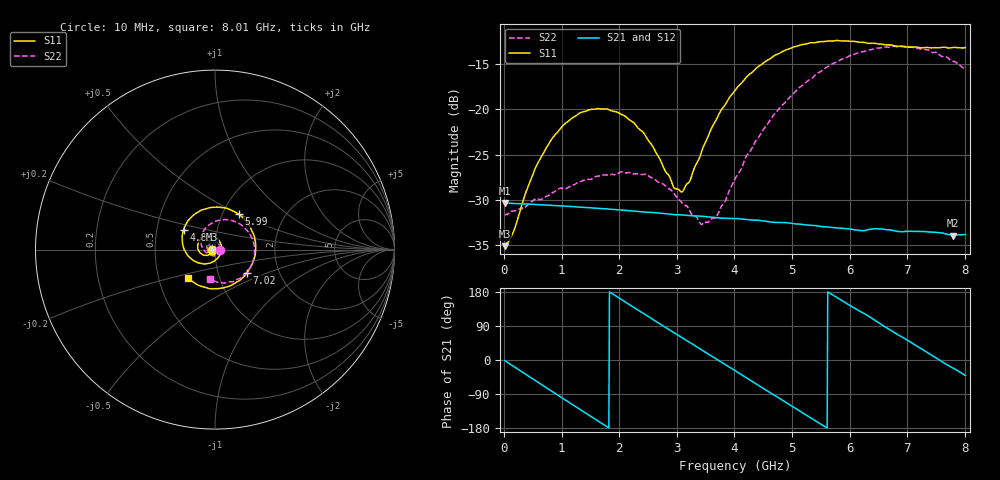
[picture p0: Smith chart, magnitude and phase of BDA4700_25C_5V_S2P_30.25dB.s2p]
!Agilent Technologies,E5071B,MY42404982,A.09.10
!Date: Mon Oct 20 13:41:50 2025
!Data & Calibration Information:
!Freq	S11:SOLT2(ON)	S21:SOLT2(ON)	S12:SOLT2(ON)	S22:SOLT2(ON)
# Hz S RI R 50
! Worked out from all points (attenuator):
!   801 points, 10 MHz to 8.01 GHz, reference 50 ohm
!   highest |S21| = -30.31 dB at 10 MHz (marker M1); lowest = -33.9 dB at 7.8 GHz (marker M2)
!   lowest |S11| = -35.1 dB at 10 MHz (marker M3), VSWR 1.04, Z = 48.3 - j0.0958 ohm
!   |S11| at or under -10 dB: start of sweep to end of sweep
!   |S22| runs from -32.7 to -13.0 dB; largest |S21 - S12| = 0.00028
!   S11 on the Smith chart (normalised r, x): 10 MHz: 0.97, -0.00; 4.83 GHz: 0.69, +0.16; 5.99 GHz: 1.19, +0.50; 7.02 GHz: 1.37, -0.38; 8.01 GHz: 0.71, -0.24
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1e7  -0.0176 -0.000992  0.0305 -0.000626  0.0306 -0.000655  0.0262 -0.000837
1.5e8  -0.0185 -0.00918  0.0292 -0.00796  0.0292 -0.00794  0.0265 -0.00716
4.2e8  -0.0282 -0.025  0.0223 -0.0202  0.0223 -0.0201  0.0201 -0.0221
7e8  -0.0488 -0.0325  0.0103 -0.0279  0.0103 -0.0279  0.00599 -0.0322
1.03e9  -0.0786 -0.0223  -0.00616 -0.0287  -0.00622 -0.0286  -0.0163 -0.0327
1.35e9  -0.0962 0.00666  -0.0199 -0.0209  -0.0199 -0.0209  -0.036 -0.0178
2.09e9  -0.0495 0.0776  -0.025 0.0119  -0.0251 0.012  -0.0293 0.0339
2.68e9  0.0234 0.0496  -0.00365 0.0266  -0.00369 0.0266  0.0126 0.0376
2.95e9  0.0353 0.0111  0.00809 0.025  0.0081 0.025  0.0251 0.0235
3.1e9  0.0328 -0.0127  0.0139 0.0222  0.0138 0.0222  0.028 0.0117
3.41e9  0.00491 -0.0556  0.0226 0.0123  0.0227 0.0123  0.0205 -0.0114
3.54e9  -0.0142 -0.0689  0.0246 0.0071  0.0246 0.00709  0.0131 -0.02
3.7e9  -0.0442 -0.0779  0.0253 0.000488  0.0253 0.00046  -0.000427 -0.026
4.01e9  -0.1071 -0.0679  0.0221 -0.0117  0.0221 -0.0118  -0.0322 -0.0257
4.83e9  -0.1753 0.1109  -0.00641 -0.0229  -0.00641 -0.0229  -0.0769 0.0719
5.35e9  -0.0715 0.221  -0.0208 -0.00966  -0.0208 -0.00972  -0.0155 0.1476
5.99e9  0.1315 0.1971  -0.018 0.0125  -0.0181 0.0124  0.1284 0.1482
6.68e9  0.2255 -0.017  0.00329 0.0214  0.00334 0.0214  0.2198 0.000593
7.02e9  0.1774 -0.1307  0.0135 0.0164  0.0135 0.0164  0.2003 -0.0904
7.43e9  0.0516 -0.2118  0.0206 0.0043  0.0206 0.00439  0.1201 -0.1668
7.8e9  -0.085 -0.202  0.0187 -0.00747  0.0188 -0.00753  0.0209 -0.1828
8.01e9  -0.1488 -0.1601  0.0154 -0.0134  0.0154 -0.0134  -0.0299 -0.1625
